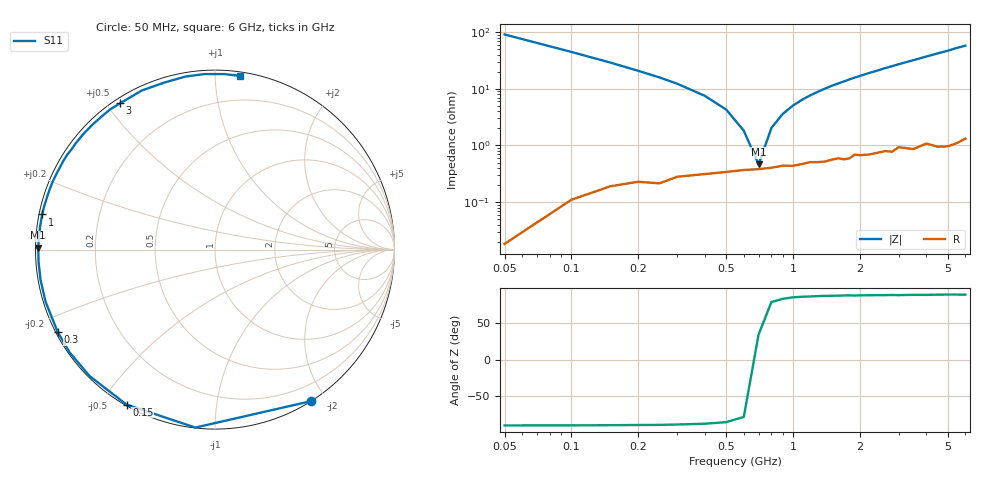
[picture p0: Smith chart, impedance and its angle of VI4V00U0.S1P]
! Infineon Technologies  Discrete & RF Semiconductors
! BB 804
! Si Tuning Diode in SOT23
! VR = 4 V
! S-Parameters:  July  1999
# GHz  S  MA  R  50
!  f  S11
! GHz  MAG  ANG
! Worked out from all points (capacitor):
!   34 points, 50 MHz to 6 GHz, reference 50 ohm
!   read as one part to ground: C = 34.8 pF near 50 MHz
!   lowest |Z| = 463 mohm at 700 MHz (marker M1)
!   series resonance near 687.2 MHz, so ESL is about 1.5 nH
!   S11 on the Smith chart (normalised r, x): 50 MHz: 0.00, -1.82; 150 MHz: 0.00, -0.58; 300 MHz: 0.01, -0.25; 1 GHz: 0.01, +0.10; 3 GHz: 0.02, +0.54; 6 GHz: 0.03, +1.15
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0.05  0.9998 -57.6
0.1  0.9976 -96.3
0.15  0.9943 -119.7
0.2  0.9922 -134.8
0.25  0.9922 -144.8
0.3  0.9895 -152.3
0.4  0.9878 -162.9
0.5  0.9865 -170.2
0.6  0.9854 -175.9
0.7  0.9848 179.4
0.8  0.984 175.4
1  0.9828 168.5
1.1  0.9816 165.4
1.3  0.9805 159.8
1.6  0.9779 152.1
1.7  0.979 149.8
1.9  0.9752 145.0
2.2  0.9761 138.5
2.4  0.9751 134.6
2.6  0.9741 130.4
2.8  0.9755 126.8
3  0.9717 123.0
3.5  0.9758 114.7
4  0.9725 106.8
4.5  0.9781 99.7
5  0.9797 93.5
5.5  0.9794 86.9
6  0.9776 81.8
